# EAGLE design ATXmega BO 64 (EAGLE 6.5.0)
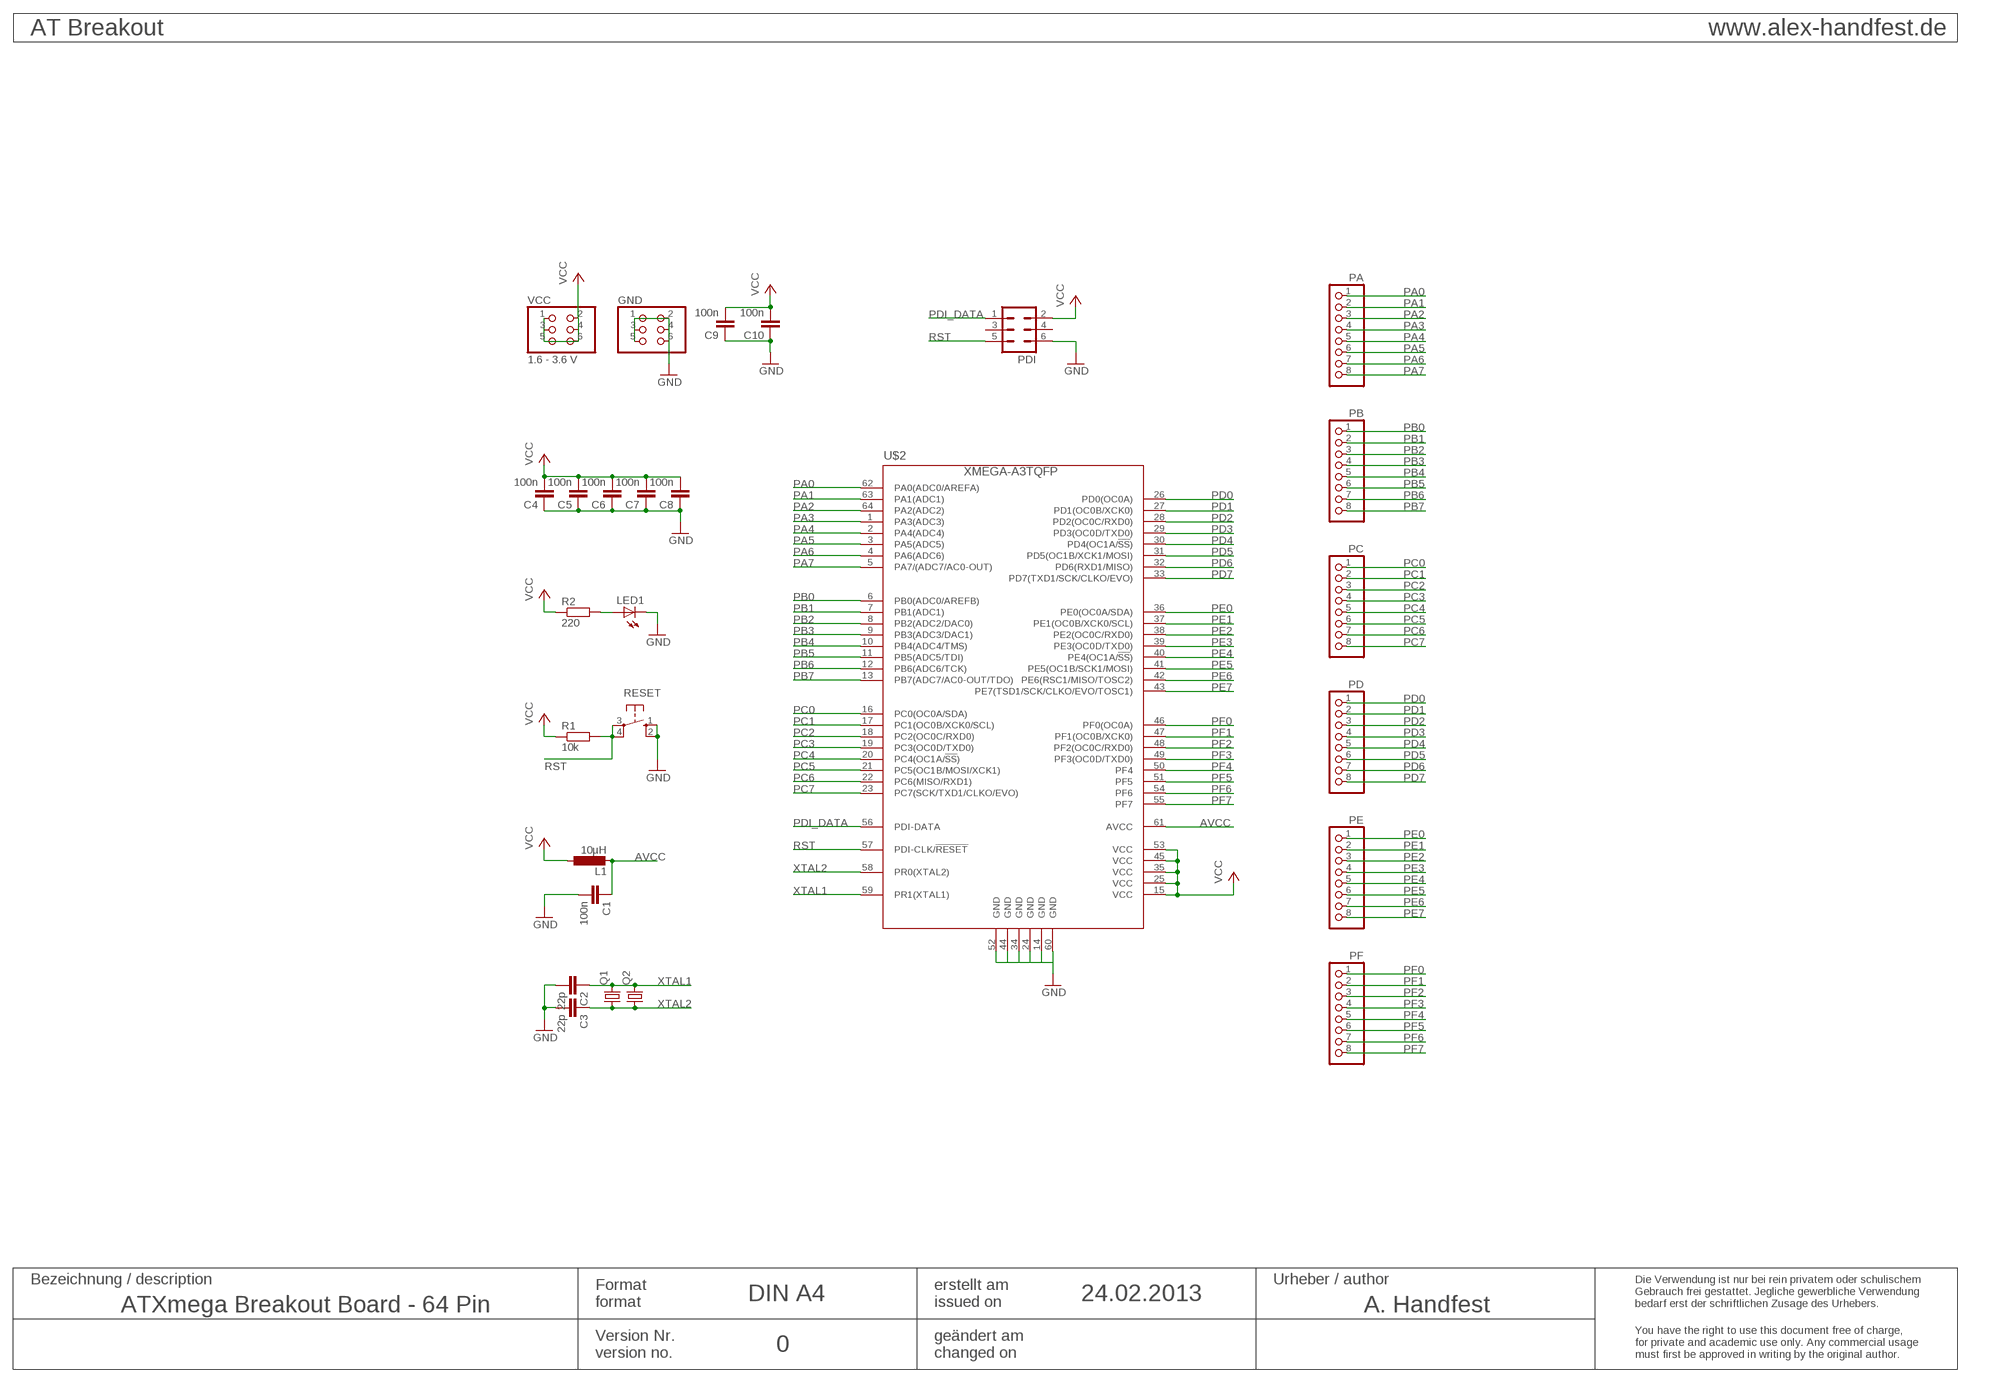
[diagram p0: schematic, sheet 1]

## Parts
C1  100n  C-EUC0805  [C0805]
C2  22p  C-EUC0805  [C0805]
C3  22p  C-EUC0805  [C0805]
C4  100n  C-EUC0805  [C0805]
C5  100n  C-EUC0805  [C0805]
C6  100n  C-EUC0805  [C0805]
C7  100n  C-EUC0805  [C0805]
C8  100n  C-EUC0805  [C0805]
C9  100n  C-EUC0805  [C0805]
C10  100n  C-EUC0805  [C0805]
GND  PINHD-2X3  [2X03]
L1  10µH  L-EUL2012C  [L2012C]
LED1  LEDCHIP-LED0805  [CHIP-LED0805]
PA  PINHD-1X8  [1X08]
PB  PINHD-1X8  [1X08]
PC  PINHD-1X8  [1X08]
PD  PINHD-1X8  [1X08]
PDI  ML6  [ML6]
PE  PINHD-1X8  [1X08]
PF  PINHD-1X8  [1X08]
Q1  CRYSTALHC49S  [HC49/S]
Q2  CRYSTALHC49UP  [HC49UP]
R1  10k  R-EU_R0805  [R0805]
R2  220  R-EU_R0805  [R0805]
RESET  10-XX  [B3F-10XX]
U$2  XMEGA-A3TQFP  [TQFP64]
VCC  1.6 - 3.6 V  PINHD-2X3  [2X03]

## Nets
AVCC: C1.1 L1.2 U$2.61(AVCC)
GND: C1.2 C2.2 C3.2 C4.1 C5.1 C6.1 C7.1 C8.1 C9.1 C10.1 GND.1 GND.2 GND.3 GND.4 GND.5 GND.6 LED1.C PDI.6 RESET.1(S) RESET.2(S1) U$2.14(GND) U$2.24(GND) U$2.34(GND) U$2.44(GND) U$2.52(GND) U$2.60(GND)
N$6: LED1.A R2.2
PA0: PA.1 U$2.62(PA0(ADC0/AREFA))
PA1: PA.2 U$2.63(PA1(ADC1))
PA2: PA.3 U$2.64(PA2(ADC2))
PA3: PA.4 U$2.1(PA3(ADC3))
PA4: PA.5 U$2.2(PA4(ADC4))
PA5: PA.6 U$2.3(PA5(ADC5))
PA6: PA.7 U$2.4(PA6(ADC6))
PA7: PA.8 U$2.5(PA7/(ADC7/AC0-OUT))
PB0: PB.1 U$2.6(PB0(ADC0/AREFB))
PB1: PB.2 U$2.7(PB1(ADC1))
PB2: PB.3 U$2.8(PB2(ADC2/DAC0))
PB3: PB.4 U$2.9(PB3(ADC3/DAC1))
PB4: PB.5 U$2.10(PB4(ADC4/TMS))
PB5: PB.6 U$2.11(PB5(ADC5/TDI))
PB6: PB.7 U$2.12(PB6(ADC6/TCK))
PB7: PB.8 U$2.13(PB7(ADC7/AC0-OUT/TDO))
PC0: PC.1 U$2.16(PC0(OC0A/SDA))
PC1: PC.2 U$2.17(PC1(OC0B/XCK0/SCL))
PC2: PC.3 U$2.18(PC2(OC0C/RXD0))
PC3: PC.4 U$2.19(PC3(OC0D/TXD0))
PC4: PC.5 U$2.20(PC4(OC1A/!SS!))
PC5: PC.6 U$2.21(PC5(OC1B/MOSI/XCK1))
PC6: PC.7 U$2.22(PC6(MISO/RXD1))
PC7: PC.8 U$2.23(PC7(SCK/TXD1/CLKO/EVO))
PD0: PD.1 U$2.26(PD0(OC0A))
PD1: PD.2 U$2.27(PD1(OC0B/XCK0))
PD2: PD.3 U$2.28(PD2(OC0C/RXD0))
PD3: PD.4 U$2.29(PD3(OC0D/TXD0))
PD4: PD.5 U$2.30(PD4(OC1A/!SS!))
PD5: PD.6 U$2.31(PD5(OC1B/XCK1/MOSI))
PD6: PD.7 U$2.32(PD6(RXD1/MISO))
PD7: PD.8 U$2.33(PD7(TXD1/SCK/CLKO/EVO))
PDI_DATA: PDI.1 U$2.56(PDI-DATA)
PE0: PE.1 U$2.36(PE0(OC0A/SDA))
PE1: PE.2 U$2.37(PE1(OC0B/XCK0/SCL))
PE2: PE.3 U$2.38(PE2(OC0C/RXD0))
PE3: PE.4 U$2.39(PE3(OC0D/TXD0))
PE4: PE.5 U$2.40(PE4(OC1A/!SS!))
PE5: PE.6 U$2.41(PE5(OC1B/SCK1/MOSI))
PE6: PE.7 U$2.42(PE6(RSC1/MISO/TOSC2))
PE7: PE.8 U$2.43(PE7(TSD1/SCK/CLKO/EVO/TOSC1))
PF0: PF.1 U$2.46(PF0(OC0A))
PF1: PF.2 U$2.47(PF1(OC0B/XCK0))
PF2: PF.3 U$2.48(PF2(OC0C/RXD0))
PF3: PF.4 U$2.49(PF3(OC0D/TXD0))
PF4: PF.5 U$2.50(PF4)
PF5: PF.6 U$2.51(PF5)
PF6: PF.7 U$2.54(PF6)
PF7: PF.8 U$2.55(PF7)
RST: PDI.5 R1.2 RESET.3(P) RESET.4(P1) U$2.57(PDI-CLK/!RESET)
VCC: C4.2 C5.2 C6.2 C7.2 C8.2 C9.2 C10.2 L1.1 PDI.2 R1.1 R2.1 U$2.15(VCC) U$2.25(VCC) U$2.35(VCC) U$2.45(VCC) U$2.53(VCC) VCC.1 VCC.2 VCC.3 VCC.4 VCC.5 VCC.6
XTAL1: C2.1 Q1.2 Q2.2 U$2.59(PR1(XTAL1))
XTAL2: C3.1 Q1.1 Q2.1 U$2.58(PR0(XTAL2))
Unconnected: PDI.3 PDI.4

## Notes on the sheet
- AT Breakout | www.alex-handfest.de
- Bezeichnung / description | Urheber / author
- Format | erstellt am
- DIN A4 | 24.02.2013
- format | issued on
- Die Verwendung ist nur bei rein privatem oder schulischem
  Gebrauch frei gestattet. Jegliche gewerbliche Verwendung 
  bedarf erst der schriftlichen Zusage des Urhebers.
- ATXmega Breakout Board - 64 Pin | A. Handfest
- Version Nr. | geändert am
- 0
- version no. | changed on
- You have the right to use this document free of charge,
  for private and academic use only. Any commercial usage
  must first be approved in writing by the original author.

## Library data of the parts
C1-C10 = rcl:C-EU: CAPACITOR, European symbol
GND VCC = pinhead:PINHD-2X3: PIN HEADER
L1 = rcl:L-EU: INDUCTOR, European symbol
LED1 = led:LED: LED
PA PB PC PD PE PF = pinhead:PINHD-1X8: PIN HEADER
PDI = con-harting-ml:ML6: HARTING
Q1 = crystal:CRYSTAL: CRYSTAL; OC_FARNELL: 1667008; OC_NEWARK: unknown
Q2 = crystal:CRYSTAL: CRYSTAL; OC_FARNELL: unknown; OC_NEWARK: unknown
R1 R2 = rcl:R-EU_: RESISTOR, European symbol
RESET = switch-omron:10-XX: OMRON SWITCH
U$2 = avr-7:XMEGA-A3: Atmel XMega A3 series processor

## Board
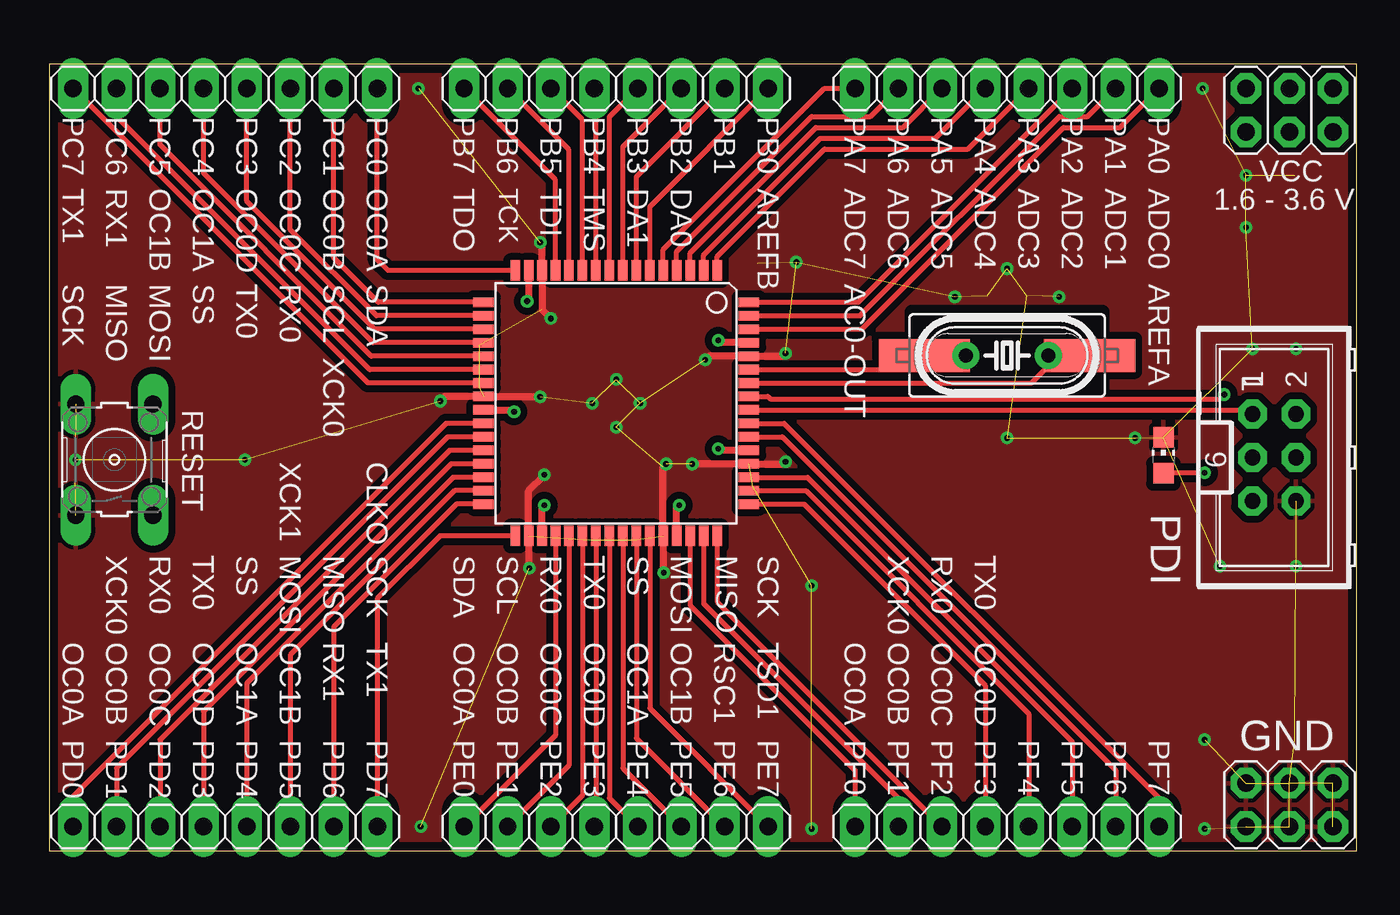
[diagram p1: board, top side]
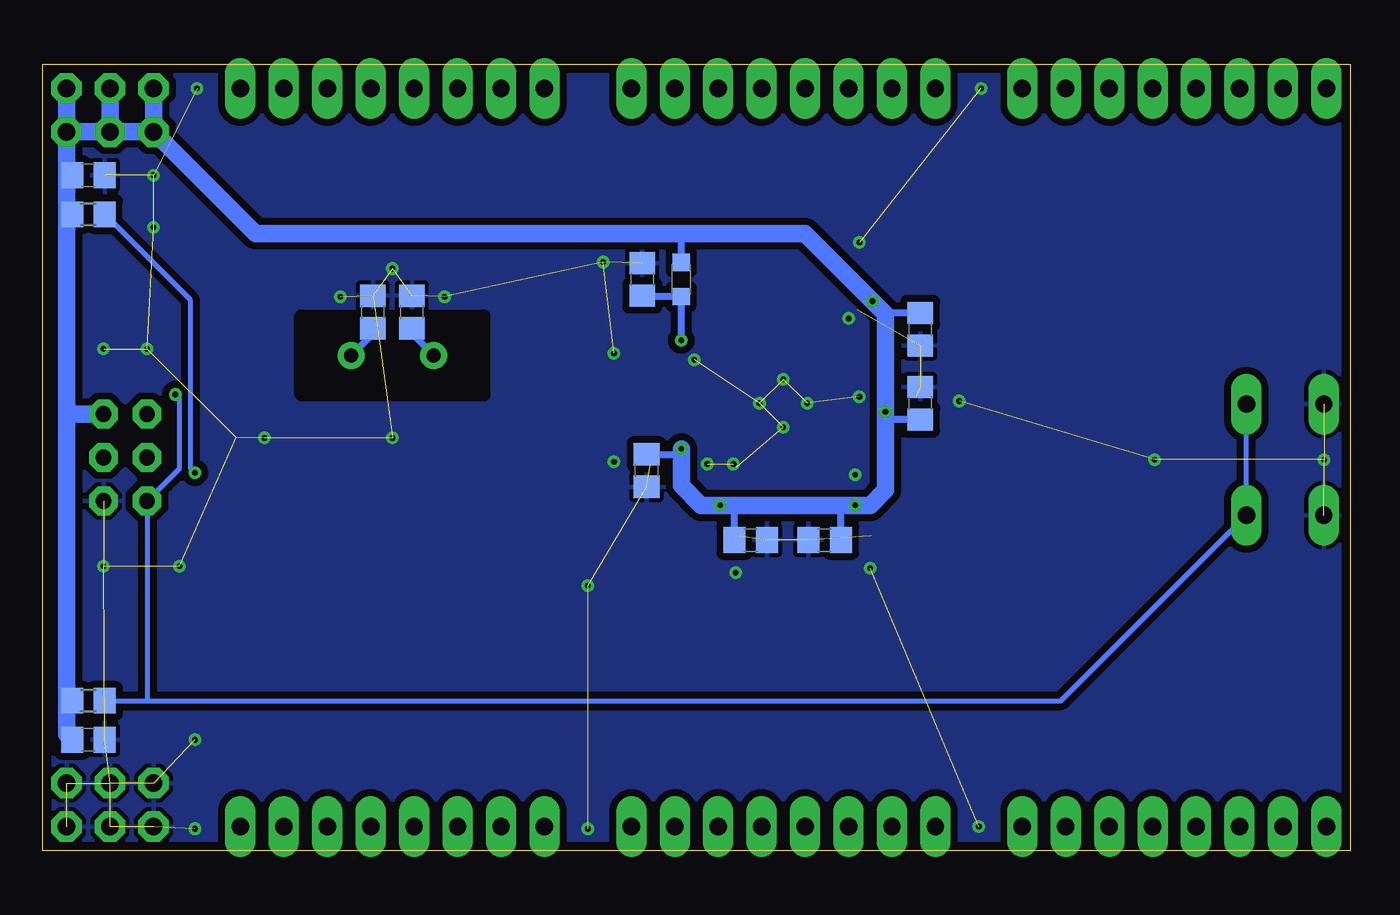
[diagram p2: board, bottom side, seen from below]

Size 76.45 x 45.97 mm. Coordinates in mm from the lower left corner, seen from the top.
Outline: 0,0 76.45,0 76.45,45.97 0,45.97 0,0
Copper layers (1*16): Top 0.035mm / dielectric 1.5mm / Bottom 0.035mm
Design rules "default *": minimum track width 10mil, minimum drill 24mil, track to track 8mil, track to pad 8mil, pad to pad 8mil, via to via 8mil, smd to smd 8mil, copper to edge 20mil, drill to drill 8mil, minimum pad ring 15mil, minimum via ring 8mil, stop-mask expansion 4mil, vias tented up to drill 20mil, thermal gap 10mil
tRestrict: area 50.4,26.4 to 61.6,31.5
bRestrict: area 50.7,26.7 to 61.3,31.2

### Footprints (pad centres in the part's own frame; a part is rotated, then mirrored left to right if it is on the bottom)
C0805 = smd 1.3 x 1.5: 1 -0.95,0; 2 0.95,0
2X03 = drill 1.016 octagon: 1 -2.54,-1.27; 2 -2.54,1.27; 3 0,-1.27; 4 0,1.27; 5 2.54,-1.27; 6 2.54,1.27
L2012C = smd 1 x 1: 1 -1,0; 2 1,0
CHIP-LED0805 = smd 1.2 x 1.2: A 0,-1.05; C 0,1.05
1X08 = drill 1.016 long: 1 -8.89,0; 2 -6.35,0; 3 -3.81,0; 4 -1.27,0; 5 1.27,0; 6 3.81,0; 7 6.35,0; 8 8.89,0
ML6 = drill 0.914 octagon: 1 -2.54,-1.27; 2 -2.54,1.27; 3 0,-1.27; 4 0,1.27; 5 2.54,-1.27; 6 2.54,1.27
HC49/S = drill 0.813: 1 -2.413,0; 2 2.413,0
HC49UP = smd 5.334 x 1.93: 1 -4.826,0; 2 4.826,0
R0805 = smd 1.3 x 1.5: 1 -0.95,0; 2 0.95,0
B3F-10XX = drill 1.016 long: 1 -3.251,2.261; 2 3.251,2.261; 3 -3.251,-2.261; 4 3.251,-2.261
TQFP64 = smd 1.194 x 0.559: 1 -7.76,5.905; 2 -7.76,5.118; 3 -7.76,4.331; 4 -7.76,3.543; 5 -7.76,2.756; 6 -7.76,1.968; 7 -7.76,1.181; 8 -7.76,0.394; 9 -7.76,-0.394; 10 -7.76,-1.181; 11 -7.76,-1.968; 12 -7.76,-2.756; 13 -7.76,-3.543; 14 -7.76,-4.331; 15 -7.76,-5.118; 16 -7.76,-5.905; 33 7.76,-5.905; 34 7.76,-5.118; 35 7.76,-4.331; 36 7.76,-3.543; 37 7.76,-2.756; 38 7.76,-1.968; 39 7.76,-1.181; 40 7.76,-0.394; 41 7.76,0.394; 42 7.76,1.181; 43 7.76,1.968; 44 7.76,2.756; 45 7.76,3.543; 46 7.76,4.331; 47 7.76,5.118; 48 7.76,5.905 | smd 0.559 x 1.194: 17 -5.905,-7.76; 18 -5.118,-7.76; 19 -4.331,-7.76; 20 -3.543,-7.76; 21 -2.756,-7.76; 22 -1.968,-7.76; 23 -1.181,-7.76; 24 -0.394,-7.76; 25 0.394,-7.76; 26 1.181,-7.76; 27 1.968,-7.76; 28 2.756,-7.76; 29 3.543,-7.76; 30 4.331,-7.76; 31 5.118,-7.76; 32 5.905,-7.76; 49 5.905,7.76; 50 5.118,7.76; 51 4.331,7.76; 52 3.543,7.76; 53 2.756,7.76; 54 1.968,7.76; 55 1.181,7.76; 56 0.394,7.76; 57 -0.394,7.76; 58 -1.181,7.76; 59 -1.968,7.76; 60 -2.756,7.76; 61 -3.543,7.76; 62 -4.331,7.76; 63 -5.118,7.76; 64 -5.905,7.76

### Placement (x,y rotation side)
C1  41.4,33.4 90 bottom
C2  54.86,31.5 90 bottom
C3  57.15,31.5 90 bottom
C4  25.15,30.48 90 bottom
C5  25.15,26.16 270 bottom
C6  30.73,18.16 0 bottom
C7  35.05,18.16 180 bottom
C8  41.15,22.23 90 bottom
C9  73.79,6.48 180 bottom
C10  73.79,39.5 180 bottom
GND  72.52,2.67 0 top
L1  39.12,33.4 270 bottom
LED1  65.15,23.11 0 top
PA  56.01,44.58 180 top
PB  33.15,44.58 180 top
PC  10.29,44.58 180 top
PD  10.29,1.4 0 top
PDI  71.63,22.99 270 top
PE  33.15,1.4 0 top
PF  56.01,1.4 0 top
Q1  56.01,28.96 180 top
Q2  56.01,28.96 180 top
R1  73.79,8.76 0 bottom
R2  73.79,37.21 0 bottom
RESET  3.81,22.86 90 top
U$2  33.15,26.16 270 top
VCC  72.52,43.31 0 top

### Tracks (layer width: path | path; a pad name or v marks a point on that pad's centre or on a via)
AVCC  (via drill 0.33)
  Top 0.406: U$2.61 39.26,29.7 v39.12,29.84
  Bottom 0.406: v39.12,29.84 L1.2 41.35,32.4 C1.1
GND  (via drill 0.33)  (50 unrouted)
  Top 0.406: v28.07,16.51 28.03,16.55 U$2.34 28.03,21.04 v28.96,21.97 | v35.94,16.26 35.9,16.29 U$2.44 35.9,22.44 v36.07,22.61 | v43.05,22.73 42.94,22.62 U$2.52 37.6,22.62 v37.59,22.61 | v22.86,26.29 23.13,26.56 U$2.24 28.69,26.56 v28.7,26.54 | v28.7,35.56 28.82,35.45 U$2.14 28.82,31.64 v29.34,31.11 | v43.05,29.08 42.89,28.92 U$2.60 38.57,28.92 v38.35,28.7
  other vias: 1.52,22.86 31.75,26.16 33.15,27.56 34.54,26.16 33.15,24.77 59.05,32.38 52.96,32.38 56.01,34.04 43.69,34.42 63.5,24.13 72.9,16.64 68.45,16.64 72.9,29.34 70.36,29.34 69.98,39.5 69.98,36.45 67.44,44.58 21.59,44.58 11.43,22.86 21.72,1.4 44.58,1.27 67.56,1.27 67.56,6.48 56.01,24.13 44.58,15.49
  pour Bottom (isolate 0.406): -0.25,46.23 76.71,46.23 76.71,-0.25 -0.25,-0.25
  pour Top (isolate 0.406): -0.25,46.23 76.71,46.23 76.71,-0.25 -0.25,-0.25
N$6  (via drill 0.33)
  Top 0.305: LED1.A 65.19,22.1 v67.56,22.1
  Bottom 0.305: v67.56,22.1 67.82,22.35 67.82,32.19 R2.2
PA0
  Top 0.305: U$2.62 47.51,30.49 59.31,42.29 62.61,42.29 PA.1
PA1
  Top 0.305: U$2.63 47.41,31.28 59.05,42.93 60.71,42.93 PA.2
PA2
  Top 0.305: U$2.64 47.31,32.07 PA.3
PA3
  Top 0.305: U$2.1 39.05,34.73 45.34,41.02 53.72,41.02 PA.4
PA4
  Top 0.305: U$2.2 38.27,34.84 45.09,41.66 51.82,41.66 PA.5
PA5
  Top 0.305: U$2.3 37.48,34.94 44.83,42.29 49.91,42.29 PA.6
PA6
  Top 0.305: U$2.4 36.69,35.04 44.58,42.93 48.01,42.93 PA.7
PA7
  Top 0.305: U$2.5 35.9,35.14 45.34,44.58 PA.8
PB0
  Top 0.305: U$2.6 35.12,37.66 PB.1
PB1
  Top 0.305: U$2.7 34.33,39.41 PB.2
PB2
  Top 0.305: U$2.8 33.54,41.16 PB.3
PB3
  Top 0.305: U$2.9 32.75,42.91 PB.4
PB4
  Top 0.305: U$2.10 31.97,44.49 PB.5
PB5
  Top 0.305: U$2.11 31.18,42.74 PB.6
PB6
  Top 0.305: U$2.12 30.39,40.98 PB.7
PB7
  Top 0.305: U$2.13 29.6,39.23 PB.8
PC0
  Top 0.305: U$2.16 19.8,33.92 19.18,34.54 PC.1
PC1
  Top 0.305: U$2.17 19.24,32.07 16.64,34.67 PC.2
PC2
  Top 0.305: U$2.18 19.14,31.28 14.1,36.32 PC.3
PC3
  Top 0.305: U$2.19 19.04,30.49 11.56,37.97 PC.4
PC4
  Top 0.305: U$2.20 18.94,29.7 9.02,39.62 PC.5
PC5
  Top 0.305: U$2.21 18.83,28.92 6.48,41.27 PC.6
PC6
  Top 0.305: U$2.22 18.73,28.13 3.94,42.93 PC.7
PC7
  Top 0.305: U$2.23 18.63,27.34 PC.8
PD0
  Top 0.305: U$2.26 23.2,24.98 1.4,3.17 PD.1
PD1
  Top 0.305: U$2.27 23.3,24.19 3.94,4.83 PD.2
PD2
  Top 0.305: U$2.28 23.41,23.41 6.48,6.48 PD.3
PD3
  Top 0.305: U$2.29 23.51,22.62 9.02,8.13 PD.4
PD4
  Top 0.305: U$2.30 23.61,21.83 11.56,9.78 PD.5
PD5
  Top 0.305: U$2.31 23.71,21.04 14.1,11.43 PD.6
PD6
  Top 0.305: U$2.32 23.81,20.26 16.64,13.08 PD.7
PD7
  Top 0.305: U$2.33 22.85,18.4 19.18,14.73 PD.8
PDI_DATA
  Top 0.305: U$2.56 70.12,25.77 PDI.1
PE0
  Top 0.305: U$2.36 29.6,6.74 PE.1
PE1
  Top 0.305: U$2.37 30.39,4.99 PE.2
PE2
  Top 0.305: U$2.38 31.18,3.24 PE.3
PE3
  Top 0.305: U$2.39 31.97,1.49 PE.4
PE4
  Top 0.305: U$2.40 32.75,3.06 PE.5
PE5
  Top 0.305: U$2.41 33.54,4.81 PE.6
PE6
  Top 0.305: U$2.42 34.33,6.57 PE.7
PE7
  Top 0.305: U$2.43 35.12,8.32 PE.8
PF0
  Top 0.305: U$2.46 37.48,14.34 47.12,4.7 PF.1
PF1
  Top 0.305: U$2.47 38.27,14.44 49.66,3.05 PF.2
PF2
  Top 0.305: U$2.48 39.05,14.54 PF.3
PF3
  Top 0.305: U$2.49 44.13,20.26 54.74,9.65 PF.4
PF4
  Top 0.305: U$2.50 44.23,21.04 57.28,8 PF.5
PF5
  Top 0.305: U$2.51 44.34,21.83 59.82,6.35 PF.6
PF6
  Top 0.305: U$2.54 42.86,24.19 62.36,4.7 PF.7
PF7
  Top 0.305: U$2.55 42.96,24.98 64.9,3.05 PF.8
RST  (via drill 0.33)
  Top 0.305: U$2.57 42.02,26.56 42.16,26.42 68.45,26.42 v68.71,26.67
  Bottom 0.305: v68.71,26.67 68.45,26.42 68.45,22.35 PDI.5 70.36,8.76 | R1.2 70.36,8.76 | 70.36,8.76 16.92,8.76 RESET.3 RESET.4
VCC  (via drill 0.33)
  Top 0.406: U$2.45 36.69,20.05 v36.83,20.19 | U$2.53 39.2,23.41 v39.12,23.5 | U$2.35 28.82,20.05 v28.96,20.19 | U$2.25 27.06,25.77 v27.18,25.65 | U$2.15 28.03,32.22 v27.94,32.13
  Bottom 0.406: R1.1 75.06,8.76 | C10.2 75.06,39.5 | R2.1 75.06,37.21 | C4.2 27.12,31.43 27.18,31.37 | C5.2 27.11,25.21 27.18,25.15 | C6.2 29.78,20.13 29.72,20.19 | C7.2 36,20.13 36.07,20.19 | C8.2 39.44,23.18 v39.12,23.5 | L1.1 39.12,36.07
  Bottom 1.016: VCC.5 75.06,39.5 75.06,37.21 75.06,25.53 | 75.06,25.53 75.06,8.76 75.06,6.8 C9.2 | PDI.2 75.06,25.53 | v39.12,23.5 39.12,21.34 37.97,20.19 v36.83,20.19 36.07,20.19 29.72,20.19 v28.96,20.19 28.07,20.19 27.18,21.08 27.18,25.15 v27.18,25.65 27.18,31.37 v27.94,32.13 31.88,36.07 39.12,36.07 64.01,36.07 VCC.1 | VCC.1 VCC.3 | VCC.3 VCC.5 | VCC.6 VCC.5 | VCC.4 VCC.3 | VCC.2 VCC.1
XTAL1
  Top 0.305: U$2.59 50.35,28.13 Q2.2 Q1.2
  Bottom 0.406: C2.1 54.86,30.23 Q1.2
XTAL2
  Top 0.305: U$2.58 57.44,27.34 58.42,28.32 Q1.1 Q2.1
  Bottom 0.406: C3.1 57.15,30.23 Q1.1

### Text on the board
tNames: PC7 | PC6 | PC5 | PC4 | PC3 | PC2 | PC1 | PC0 | PB7 | PB6 | PB5 | PB4 | PB3 | PB2 | PB1 | PB0 | PA7 | PA6 | PA5 | PA4 | PA3 | PA2 | PA1 | PA0 | TX1 | RX1 | OC1B | OC1A | OC0D | OC0C | OC0B | OC0A | TDO | TCK | TDI | TMS | DA1 | DA0 | AREFB | ADC7 | ADC6 | ADC5 | ADC4 | ADC3 | ADC2 | ADC1 | ADC0 | SCK | MISO | MOSI | SS | TX0 | RX0 | SCL | SDA | AC0-OUT | AREFA | XCK0 | 1 | XCK1 | CLKO | XCK0 | RX0 | TX0 | SS | MOSI | MISO | SCK | SDA | SCL | RX0 | TX0 | SS | MOSI | MISO | SCK | XCK0 | RX0 | TX0 | OC0A | OC0B | OC0C | OC0D | OC1A | OC1B | RX1 | TX1 | OC0A | OC0B | OC0C | OC0D | OC1A | OC1B | RSC1 | TSD1 | OC0A | OC0B | OC0C | OC0D | PD0 | PD1 | PD2 | PD3 | PD4 | PD5 | PD6 | PD7 | PE0 | PE1 | PE2 | PE3 | PE4 | PE5 | PE6 | PE7 | PF0 | PF1 | PF2 | PF3 | PF4 | PF5 | PF6 | PF7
